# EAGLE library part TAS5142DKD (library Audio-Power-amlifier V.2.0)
The TAS5142 is a third-generation, high-performance, integrated stereo digital amplifier power stage with an improved protection system. The TAS5142 is capable of driving a 4-W bridge-tied load (BTL) at up to 100 W per channel with low integrated noise at the output, low THD+N performance, and low idle power dissipation.
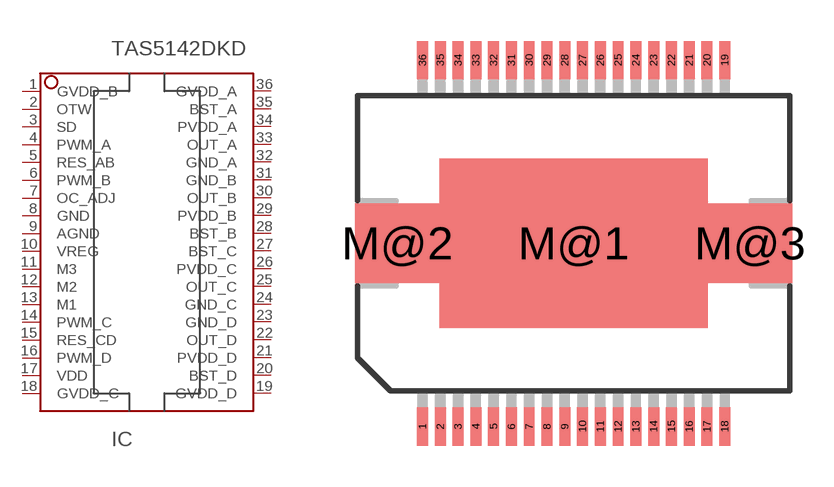
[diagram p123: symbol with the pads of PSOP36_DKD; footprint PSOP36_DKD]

Designator prefix IC

## TAS5142DKD  [PSOP36_DKD]
1  GVDD_B
2  OTW  out
3  SD  out
4  PWM_A  in
5  RES_AB  in
6  PWM_B  in
7  OC_ADJ  out
8  GND  pwr
9  AGND  pwr
10  VREG  pwr
11  M3  in
12  M2  in
13  M1  in
14  PWM_C  in
15  RES_CD  in
16  PWM_D  in
17  VDD  pwr
18  GVDD_C  pwr
19  GVDD_D  pwr
20  BST_D  pwr
21  PVDD_D  pwr
22  OUT_D  out
23  GND_D  pwr
24  GND_C  pwr
25  OUT_C  out
26  PVDD_C  pwr
27  BST_C  pwr
28  BST_B  pwr
29  PVDD_B  pwr
30  OUT_B  out
31  GND_B  pwr
32  GND_A  pwr
33  OUT_A  out
34  PVDD_A  pwr
35  BST_A  pwr
36  GVDD_A  pwr

## Footprint PSOP36_DKD (pad centres in mm)
36-Lead Power Small Ou t l i ne Package ( P S O P ) , s i m i l a r t o JEDEC out l i ne MO- 1 6 6 , var i a t i on AE:f
smd 0.4 x 1.4: 1 -5.525,-6.7; 2 -4.875,-6.7; 3 -4.225,-6.7; 4 -3.575,-6.7; 5 -2.925,-6.7; 6 -2.275,-6.7; 7 -1.625,-6.7; 8 -0.975,-6.7; 9 -0.325,-6.7; 10 0.325,-6.7; 11 0.975,-6.7; 12 1.625,-6.7; 13 2.275,-6.7; 14 2.925,-6.7; 15 3.575,-6.7; 16 4.225,-6.7; 17 4.875,-6.7; 18 5.525,-6.7; 19 5.525,6.7; 20 4.875,6.7; 21 4.225,6.7; 22 3.575,6.7; 23 2.925,6.7; 24 2.275,6.7; 25 1.625,6.7; 26 0.975,6.7; 27 0.325,6.7; 28 -0.325,6.7; 29 -0.975,6.7; 30 -1.625,6.7; 31 -2.275,6.7; 32 -2.925,6.7; 33 -3.575,6.7; 34 -4.225,6.7; 35 -4.875,6.7; 36 -5.525,6.7
smd 9.8 x 6.2: M@1 0,0
smd 3.1 x 2.9: M@2 -6.45,0; M@3 6.45,0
